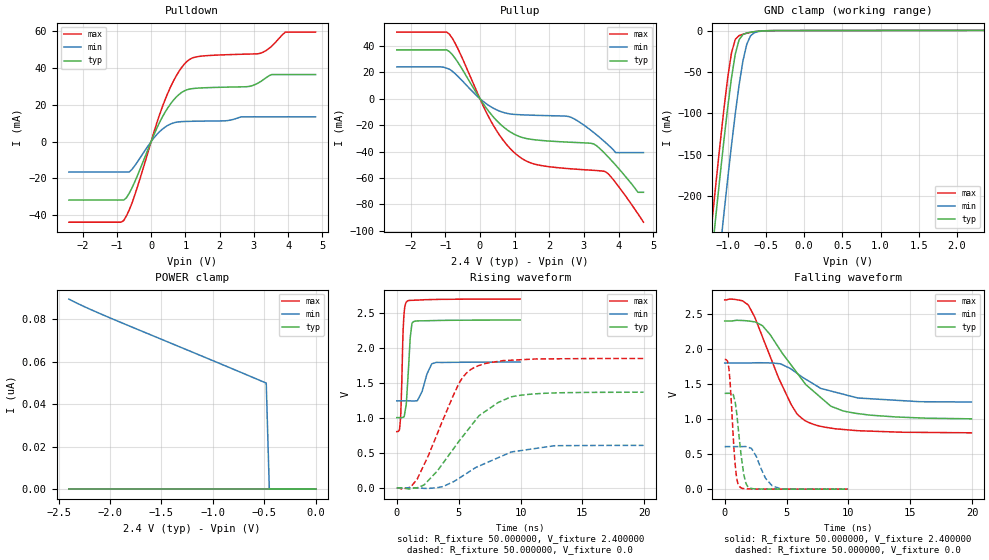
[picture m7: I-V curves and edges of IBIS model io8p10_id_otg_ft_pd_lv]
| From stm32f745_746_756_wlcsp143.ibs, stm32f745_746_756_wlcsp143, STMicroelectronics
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|   Model io8p10_id_otg_ft_pd_lv
[Model]  io8p10_id_otg_ft_pd_lv
Model_type I/O
Polarity   Non-Inverting
Enable   Active-Low
Vinl =   0.720000V
Vinh =   1.680000V
Vmeas =  1.200000V
Cref =   40.000000pF
Rref =   100.000000M
Vref =   0.0V
C_comp   2.229800pF   2.169700pF   2.325100pF
[Temperature Range]   25.000000   0.125000k   -40.000000
[Pullup Reference]   2.400000V   1.800000V   2.700000V
[Pulldown Reference]   0.0V   0.0V   0.0V
[POWER Clamp Reference]   2.400000V   1.800000V   2.700000V
[GND Clamp Reference]   0.0V   0.0V   0.0V
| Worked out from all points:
|   slope of the pulldown table from 0 to 0.36 V, typ, clamps not added: 25 ohm
|   slope of the pullup table from 0 to 0.36 V, typ, clamps not added: 27.7 ohm
|   GND clamp passes 1 mA (typ) near -0.62 V on its own axis
|   rising waveform, R_fixture 50.000000, V_fixture 2.400000: 20-80 % time 278ps typ, 621ps min, 185ps max; typ from 1 V to 2.4 V
|   rising waveform, R_fixture 50.000000, V_fixture 0.0: 20-80 % time 3.75ns typ, 4.02ns min, 2.67ns max; typ from 0 V to 1.37 V
|   falling waveform, R_fixture 50.000000, V_fixture 2.400000: 20-80 % time 3.94ns typ, 4.01ns min, 2.73ns max; typ from 2.4 V to 1 V
|   falling waveform, R_fixture 50.000000, V_fixture 0.0: 20-80 % time 528ps typ, 975ps min, 382ps max; typ from 1.37 V to 0 V
[Pulldown]
|Voltage   I(typ)   I(min)   I(max)
-2.4V     -31.73mA   -16.51mA   -43.74mA
-800mV    -31.73mA   -16.51mA   -42.87mA
-480mV    -21.97mA   -13.17mA   -29.2mA
80mV      3.629mA    1.966mA    5.013mA
480mV     18.15mA    8.737mA    26.01mA
800mV     25.37mA    10.71mA    37.77mA
1.12V     28.53mA    11.02mA    44.6mA
2.8V      29.83mA    13.48mA    47.51mA
3.2V      32.64mA    13.48mA    48.03mA
3.52V     36.41mA    13.48mA    51.82mA
3.92V     36.41mA    13.48mA    59.47mA
4.8V      36.41mA    13.48mA    59.47mA
[Pullup]
|Voltage   I(typ)   I(min)   I(max)
-2.4V     36.9mA     24.03mA    50.36mA
-960mV    36.9mA     23.04mA    50.36mA
-640mV    27.65mA    17.03mA    37.99mA
320mV     -11.75mA   -6.207mA   -17.08mA
960mV     -26.47mA   -11.82mA   -40.02mA
1.52V     -30.88mA   -12.51mA   -49.05mA
2.56V     -32.88mA   -13.48mA   -52.9mA
3.28V     -34.19mA   -25.52mA   -54.18mA
3.6V      -41.31mA   -32.62mA   -54.98mA
3.92V     -50.33mA   -40.8mA    -63.62mA
4.56V     -70.8mA    -40.8mA    -87.07mA
4.72V     -70.8mA    -40.8mA    -93.4mA
[GND_clamp]
|Voltage   I(typ)   I(min)   I(max)
-2.4V     -1.424A    -1.508A    -1.393A
-1.25V    -311.2mA   -401.9mA   -273.3mA
-1.2V     -265.4mA   -356.1mA   -227.2mA
-1.15V    -220.4mA   -310.8mA   -181.9mA
-1.1V     -176.3mA   -266.2mA   -137.9mA
-1.05V    -133.8mA   -222.5mA   -95.89mA
-950mV    -57.33mA   -138.9mA   -27.03mA
-900mV    -28.31mA   -100.4mA   -10.67mA
-850mV    -11.07mA   -65.56mA   -6.047mA
-750mV    -2.904mA   -16.55mA   -3.26mA
-600mV    -808.2uA   -1.212mA   -806.8uA
2.35V     242.6uA    152uA      283.9uA
[POWER_clamp]
|Voltage   I(typ)   I(min)   I(max)
-2.4V     0A         89.62nA    0A
-2.04V    0A         81.58nA    0A
-480mV    0A         50.01nA    0A
-450mV    0A         0A         0A
0V        0A         0A         0A
[Ramp]
| variable   typ   min   max
dV/dt_r  0.81942/3.74550n   0.36445/4.02212n   1.11090/2.67986n
dV/dt_f  0.83334/3.93761n   0.33360/4.08325n   1.13504/2.73520n
R_load = 50.000000
[Rising Waveform]
R_fixture= 50.000000
V_fixture= 2.400000
V_fixture_min= 1.800000
V_fixture_max= 2.700000
|time   V(typ)   V(min)   V(max)
0s        1.003V     1.242V     802.8mV
220.2ps   1.003V     1.242V     829.3mV
300.3ps   1.002V     1.242V     987.1mV
560.6ps   1.011V     1.242V     2.419V
820.8ps   1.342V     1.242V     2.661V
1.081ns   2.13V      1.242V     2.676V
1.341ns   2.371V     1.24V      2.678V
2.042ns   2.384V     1.374V     2.684V
2.843ns   2.388V     1.772V     2.688V
9.97ns    2.396V     1.796V     2.695V
[Rising Waveform]
R_fixture= 50.000000
V_fixture= 0.0
V_fixture_min= 0.0
V_fixture_max= 0.0
|time   V(typ)   V(min)   V(max)
0s        168.9uV    66.49uV    586.3uV
1.121ns   -14.72mV   125.1uV    12.37mV
1.642ns   550.7uV    -515.2uV   121.8mV
3.283ns   241.9mV    2.477mV    777.3mV
5.005ns   660.4mV    134.3mV    1.485V
6.246ns   939.8mV    275mV      1.716V
8.168ns   1.215V     428.3mV    1.805V
9.57ns    1.31V      520.6mV    1.825V
12.77ns   1.355V     601.6mV    1.842V
19.94ns   1.366V     606.5mV    1.847V
[Falling Waveform]
R_fixture= 50.000000
V_fixture= 2.400000
V_fixture_min= 1.800000
V_fixture_max= 2.700000
|time   V(typ)   V(min)   V(max)
0s        2.396V     1.796V     2.695V
1.441ns   2.403V     1.796V     2.683V
1.922ns   2.395V     1.797V     2.619V
3.083ns   2.322V     1.8V       2.156V
4.364ns   2.015V     1.788V     1.581V
5.365ns   1.769V     1.712V     1.209V
6.527ns   1.496V     1.568V     973.5mV
8.569ns   1.183V     1.399V     870.2mV
9.85ns    1.104V     1.34V      846.4mV
19.94ns   1.003V     1.242V     802.8mV
[Falling Waveform]
R_fixture= 50.000000
V_fixture= 0.0
V_fixture_min= 0.0
V_fixture_max= 0.0
|time   V(typ)   V(min)   V(max)
0s        1.366V     606.5mV    1.847V
340.3ps   1.366V     606.5mV    1.715V
440.4ps   1.365V     606.5mV    1.517V
700.7ps   1.341V     606.4mV    720.6mV
940.9ps   1.122V     606.1mV    194.5mV
1.221ns   652.9mV    606mV      33.76mV
1.542ns   213.2mV    607.1mV    7.476mV
2.022ns   17.93mV    589.9mV    2.845mV
3.844ns   1.249mV    47.82mV    1.395mV
9.97ns    168.9uV    66.49uV    586.3uV
